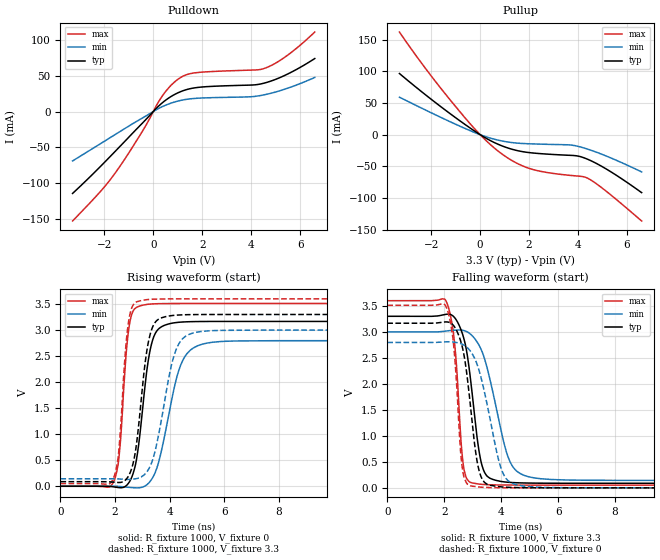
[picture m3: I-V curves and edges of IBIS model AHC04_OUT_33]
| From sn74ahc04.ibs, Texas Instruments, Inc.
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[Model]   AHC04_OUT_33
Model_type  Output
Vref =   0
Rref =   1000
Cref =   50p
Vmeas =   1.65
| variable   typ   min   max
C_comp   2.86pF   1.54pF   4.00pF
| C_pullup   2.82pF   1.54pF   3.49pF
| C_pulldown   2.90pF   1.77pF   4.00pF
[Temperature Range]   40   100   -40
| Ambient temperature   25   85   -40
[Voltage range]   3.3   3   3.6
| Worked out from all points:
|   slope of the pulldown table from 0 to 0.495 V, typ, clamps not added: 31.8 ohm
|   slope of the pullup table from 0 to 0.495 V, typ, clamps not added: 45.8 ohm
|   rising waveform, R_fixture 1000, V_fixture 0: 20-80 % time 434ps typ, 700ps min, 283ps max; typ from 0 V to 3.17 V
|   falling waveform, R_fixture 1000, V_fixture 3.3: 20-80 % time 439ps typ, 727ps min, 267ps max; typ from 3.3 V to 0.088 V
|   rising waveform, R_fixture 1000, V_fixture 3.3: 20-80 % time 418ps typ, 632ps min, 279ps max; typ from 0.088 V to 3.3 V
|   falling waveform, R_fixture 1000, V_fixture 0: 20-80 % time 419ps typ, 665ps min, 255ps max; typ from 3.17 V to 0 V
[Pulldown]
| AHC04_OUT_33
|   Voltage   I(typ)   I(min)   I(max)
-3.3V     -114.4mA   -69.04mA   -152.9mA
-2.22V    -78.8mA    -46.22mA   -113.9mA
-1.635V   -58.39mA   -33.79mA   -89.51mA
-480mV    -17.44mA   -9.793mA   -29.54mA
330mV     11.04mA    6.164mA    19.74mA
635mV     18.98mA    10.63mA    33.32mA
955mV     25.27mA    14.14mA    43.64mA
1.295V    29.94mA    16.67mA    50.63mA
1.685V    33.04mA    18.27mA    53.93mA
4.555V    39.87mA    23.49mA    60.41mA
5.45V     51.66mA    32.05mA    77.66mA
6.6V      73.99mA    47.56mA    111mA
[Pullup]
| AHC04_OUT_33
|   Voltage   I(typ)   I(min)   I(max)
-3.3V     96.43mA    59.11mA    161.8mA
-2.19V    61.53mA    38.04mA    102.2mA
-995mV    26.52mA    16.31mA    43.97mA
-15mV     367.5uA    219.4uA    603.7uA
745mV     -15.3mA    -8.685mA   -26.19mA
1.415V    -24.13mA   -12.91mA   -43.25mA
2.085V    -28.58mA   -14.44mA   -54.08mA
3.69V     -32.57mA   -16.26mA   -64.18mA
4.03V     -33.95mA   -18.66mA   -65.36mA
4.39V     -38.7mA    -22.73mA   -68.57mA
5.315V    -57.85mA   -36.24mA   -94.18mA
6.6V      -91.36mA   -58.68mA   -136.1mA
[Ramp]
| AHC04_OUT_33
| variable   typ   min   max
dV/dt_r   1.92/4.43E-10   1.70/7.09E-10   2.12/2.98E-10
dV/dt_f   1.95/4.54E-10   1.74/7.41E-10   2.15/2.80E-10
R_load = 1000
[Rising Waveform]
| AHC04_OUT_33
R_fixture =   1000
C_fixture =   0
L_fixture =   0
V_fixture =   0
V_fixture_min = 0
V_fixture_max = 0
|   Time   V(typ)   V(min)   V(max)
0s        923.7pV    1.562nV    526.1pV
1.94ns    -10.94mV   922.7uV    79.68mV
2.15ns    -26.28mV   -3.1mV     589.2mV
2.545ns   101.3mV    -22.73mV   3.159V
2.815ns   610.7mV    -30.5mV    3.445V
3.155ns   2.186V     25.06mV    3.492V
3.53ns    2.984V     346.5mV    3.507V
4.465ns   3.155V     2.401V     3.511V
5.6ns     3.166V     2.769V     3.511V
50ns      3.167V     2.797V     3.511V
[Falling Waveform]
| AHC04_OUT_33
R_fixture =   1000
C_fixture =   0
L_fixture =   0
V_fixture =   3.3
V_fixture_min = 3
V_fixture_max = 3.6
|   Time   V(typ)   V(min)   V(max)
0s        3.3V       3V         3.6V
2.07ns    3.338V     3.017V     3.585V
2.355ns   3.28V      3.033V     2.824V
2.595ns   3.032V     3.034V     858.1mV
2.69ns    2.869V     3.026V     367.8mV
3.225ns   698.1mV    2.74V      73.16mV
3.51ns    222.2mV    2.3V       61.01mV
4.31ns    104.6mV    504mV      53.79mV
5.385ns   89.79mV    175.3mV    52.7mV
50ns      87.98mV    143.4mV    52.56mV
[Rising Waveform]
| AHC04_OUT_33
R_fixture =   1000
C_fixture =   0
L_fixture =   0
V_fixture =   3.3
V_fixture_min = 3
V_fixture_max = 3.6
|   Time   V(typ)   V(min)   V(max)
0s        87.98mV    143.4mV    52.56mV
1.925ns   79.6mV     143.7mV    133.8mV
2.13ns    72.37mV    140.4mV    638.1mV
2.52ns    223.7mV    131.9mV    3.237V
2.765ns   732.8mV    144.8mV    3.534V
3.115ns   2.421V     243.6mV    3.582V
3.465ns   3.144V     673.1mV    3.595V
4.235ns   3.287V     2.622V     3.6V
5.2ns     3.299V     2.976V     3.6V
50ns      3.3V       3V         3.6V
[Falling Waveform]
| AHC04_OUT_33
R_fixture =   1000
C_fixture =   0
L_fixture =   0
V_fixture =   0
V_fixture_min = 0
V_fixture_max = 0
|   Time   V(typ)   V(min)   V(max)
0s        3.167V     2.797V     3.511V
2.065ns   3.192V     2.809V     3.483V
2.325ns   3.123V     2.805V     2.775V
2.63ns    2.718V     2.763V     398.7mV
3ns       1.167V     2.561V     30.42mV
3.15ns    523.1mV    2.382V     20.62mV
3.315ns   186.7mV    2.071V     12.06mV
4.04ns    17.32mV    313.1mV    1.945mV
4.905ns   2.668mV    27.01mV    339uV
50ns      -13.44nV   -7.509nV   -6.235nV
